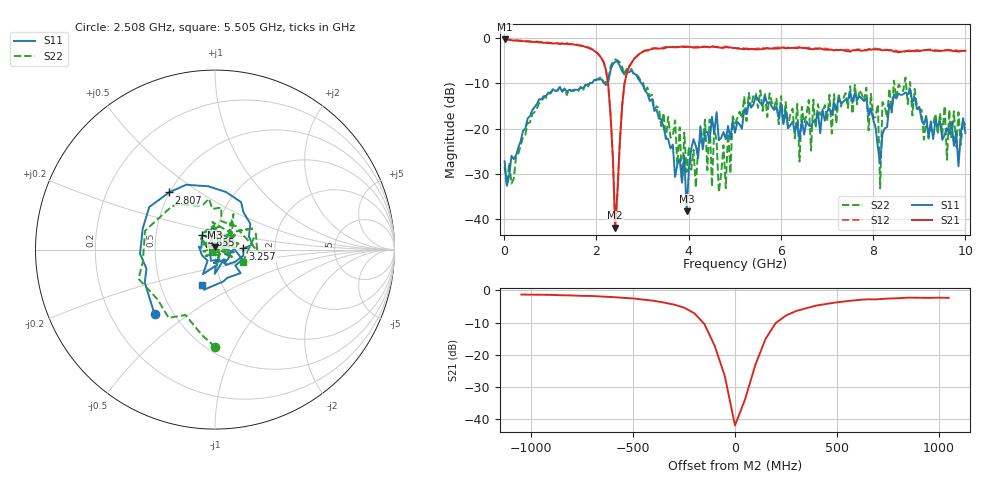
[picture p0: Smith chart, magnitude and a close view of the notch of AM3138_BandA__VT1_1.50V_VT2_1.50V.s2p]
! Date/Time: Tue, Nov 13, 2018 4:42 PM
! Network Analyzer: Agilent Technologies E8364B Rev: A.07.50.67
! Sweep from 0.010 to 10.000 GHz, 201 Points, Sweep Type: LIN
! Power Supply: 1.501 V, 0.000 A
# Hz S DB R 50
!freq MagS11 AngS11 MagS21 AngS21 MagS12 AngS12 MagS22 AngS22
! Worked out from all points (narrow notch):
!   201 points, 10 MHz to 10 GHz, reference 50 ohm
!   highest |S21| = -0.24 dB at 10 MHz (marker M1); lowest = -41.9 dB at 2.408 GHz (marker M2)
!   notch at M2: 39.5 dB deep, 180 MHz wide at half that depth
!   lowest |S11| = -38.3 dB at 3.956 GHz (marker M3), VSWR 1.02, Z = 50.1 + j1.22 ohm
!   |S11| at or under -10 dB: start of sweep to 1.847 GHz; 2.18 GHz to 2.237 GHz (56.38 MHz wide, 2.55 % of centre); 2.978 GHz to end of sweep
!   |S22| runs from -34.0 to -4.7 dB; largest |S21 - S12| = 0.031
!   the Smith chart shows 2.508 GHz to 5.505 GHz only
!   S11 on the Smith chart (normalised r, x): 2.508 GHz: 0.39, -0.38; 2.807 GHz: 0.50, +0.38; 3.257 GHz: 1.37, +0.02; 4.855 GHz: 0.86, +0.14; 5.505 GHz: 0.81, -0.33
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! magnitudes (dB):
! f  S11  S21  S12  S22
! 10 MHz  -27.2  -0.2  -0.3  -28.3
! 1.708 GHz  -11.1  -1.7  -1.7  -11.7
! 2.208 GHz  -10.4  -7.1  -7.0  -9.7
! 2.408 GHz  -5.2  -41.9  -41.7  -4.7
! 2.508 GHz  -6.1  -23.1  -23.1  -5.3
! 2.807 GHz  -7.8  -4.7  -4.6  -7.8
! 3.257 GHz  -16.1  -2.3  -2.2  -15.8
! 3.357 GHz  -17.7  -2.3  -2.3  -15.5
! 3.956 GHz  -38.3  -1.9  -1.9  -29.6
! 4.106 GHz  -22.3  -2.1  -2.1  -24.7
! 4.805 GHz  -22.3  -2.0  -1.8  -33.1
! 4.855 GHz  -19.4  -2.1  -2.0  -19.9
! 5.005 GHz  -20.9  -2.2  -2.2  -18.8
! 5.505 GHz  -13.6  -2.5  -2.3  -15.4
! 6.404 GHz  -22.5  -2.1  -2.0  -27.2
! 6.703 GHz  -18.3  -2.5  -2.3  -13.6
! 7.852 GHz  -13.4  -2.7  -2.7  -10.9
! 8.102 GHz  -24.0  -2.5  -2.4  -14.6
! 8.152 GHz  -27.7  -2.5  -2.4  -33.2
! 8.202 GHz  -21.2  -2.7  -2.5  -14.2
! 8.352 GHz  -14.6  -2.7  -2.7  -11.1
! 10 GHz  -20.9  -2.8  -2.7  -19.3
